VAR_GLOBAL
	{attribute 'analysis' := '-33'}
	ipCreator: I_AcsiCodeCreatorClass := GVL_AcsiVars.Creator.SetCodeRev(codeRev:=8).SetGuiVer(major:=3, minor:=99, build:=5, revision:=0);
	
	(* IED data model *)
	{attribute 'analysis' := '-6'}
	fbIED: FB_IED_IED;
	{warning 'Please configure your server IP-address in the initialization code of the server function block below:'}
	(* Server container *)
	fbIEDServer: FB_iec61850ServerClass := (ipIED:=fbIED, settings:=(bEnable:=TRUE, sLocalHost:='127.0.0.1', nCalled_AP_InvID:=0, nCalling_AP_InvID:=0, nCalled_AE_InvID:=0, nCalling_AE_InvID:=0));
	(* Server connections *)
	fbIEDServerSession1: FB_IEDServerSession := (fbConnection:=(ipServer:=fbIEDServer, settings:=(bEnable:=TRUE)));
	(*
	fbIEDServerSession2: FB_IEDServerSession := (fbConnection:=(ipServer:=fbIEDServer, settings:=(bEnable:=TRUE)));
	...
	fbIEDServerSessionN: FB_IEDServerSession := (fbConnection:=(ipServer:=fbIEDServer, settings:=(bEnable:=TRUE)));
	*)
	
	(* Sampled values publisher *)
	fbIED_MUnn_MSVCB01SvPublisher: FB_IED_MUnn_MSVCB01SvPublisher := (fbAdapter:=(ipIED:=fbIED, settings:=(eDispatchMode:=E_GseDispatchMode.NonPromiscuous)));
	fbIED_MUnn_MSVCB02SvPublisher: FB_IED_MUnn_MSVCB02SvPublisher := (fbAdapter:=(ipIED:=fbIED, settings:=(eDispatchMode:=E_GseDispatchMode.NonPromiscuous)));
	
	(* Critical section to secure the concurrent access to IED data from multiple tasks *)
	{attribute 'analysis' := '-6'}
	fbIEDCriticalSection: FB_IecCriticalSection;
END_VAR
VAR_GLOBAL CONSTANT
	cOversampleFactor_IED_MUnn_LLN0_MSVCB02_Asdu1: UINT := 8; (* Max. number of SV oversampling ASDUs *)
END_VAR
